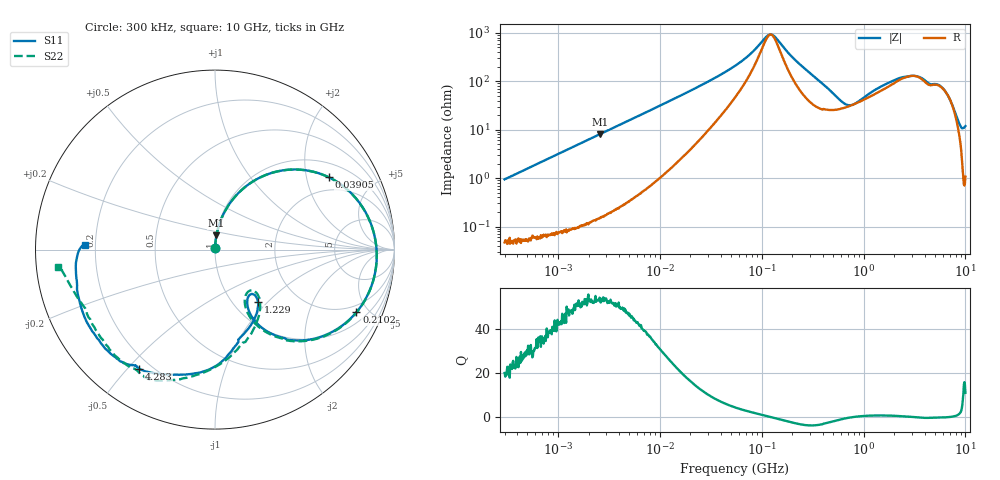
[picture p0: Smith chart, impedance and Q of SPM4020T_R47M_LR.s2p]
! S-Parameter Data Generated by TDK Corporation
! Copyright(C) 2019 TDK Corporation.
! All Rights Reserved.
! TDK P/N: SPM4020T-R47M-LR (Inductor)
! Property: L=470nH at 100kHz
! Size(LxWxT): 4.4x4.1x2mm
! Model Type: s2p (Touchstone File Format Version 1.0)
! Frequency: DC=Yes Start=0.3MHz Stop=10000MHz 802points Log-sweep
! Model Generated on Sep. 23, 2019
! Port Assignments:
!  1 ---@@@--- 2
! Applicable Conditions:
!  Temperature = 25 degC
!  DC Bias Current = 0 A
!  Small Signal Operation
! Terms and conditions regarding TDK Simulation Models
! (1)This simulation model is being provided solely for informational purposes. Please refer to the specifications of the products in terms of detailed characteristics of such products.
! (2)In no event shall TDK Corporation of any of its subsidiaries be liable for any loss or damage arising, directly or indirectly,
!  From any information contained in this simulation model, including, but not limited to loss or damages arising from any inaccuracies, omissions or errors in connection with such information.
! (3)Any and all copyrights on this simulation model are owned by TDK Corporation.
!  Duplication or redistribution of this simulation model without prior written permission from TDK Corporation is prohibited.
! (4)This simulation model is subject to any modification or change without any prior notice.
! (5)Neither TDK Corporation nor any of its subsidiaries shall make any warranty, express or implied,
!  Including but not limited to the correctness, implied warranties of merchantability and fitness for a particular purpose with respect to this simulation models.
! (6)The use of this simulation model shall be deemed to have consented to the terms and conditions hereof.
# Hz S MA R 50
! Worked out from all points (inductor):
!   801 points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, 300 kHz to 10 GHz, reference 50 ohm
!   read as one part in series: L = 498 nH near 318.3 kHz
!   highest Q = 53.8 at 2.599 MHz (marker M1), where L = 495 nH
!   self-resonance near 122.6 MHz
!   S11 on the Smith chart (normalised r, x): 300 kHz: 1.00, +0.02; 39.05 MHz: 1.47, +2.71; 210.2 MHz: 1.54, -4.19; 1.229 GHz: 1.29, -0.87; 4.283 GHz: 0.15, -0.54; 10 GHz: 0.16, +0.02
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300000  0.009137 86.2  0.9995 -0.6  0.9995 -0.5  0.009027 86.8
1713600  0.05275 85.8  0.9975 -3.1  0.9975 -3.1  0.05277 85.8
2598892  0.07965 84.2  0.9953 -4.7  0.9954 -4.7  0.07969 84.3
9671944  0.2837 71.4  0.9499 -16.8  0.95 -16.8  0.2836 71.4
2.252362e7  0.5639 50.9  0.787 -35.1  0.7871 -35.1  0.5639 50.9
3.904515e7  0.7508 32.5  0.564 -49.5  0.564 -49.5  0.7509 32.5
5.477226e7  0.8298 21.1  0.4024 -56.0  0.4024 -56.0  0.8298 21.0
1.210198e8  0.9025 -4.1  0.09762 -7.8  0.09765 -7.8  0.9025 -4.3
1.356511e8  0.9016 -7.8  0.1094 19.4  0.1095 19.4  0.9015 -8.1
2.102074e8  0.8619 -23.9  0.296 46.4  0.2961 46.4  0.8614 -24.4
3.126428e8  0.7506 -41.1  0.5083 35.0  0.5083 35.0  0.7489 -41.8
4.329008e8  0.5922 -54.4  0.6498 18.4  0.6499 18.4  0.5881 -55.3
6.242396e8  0.3991 -61.2  0.7282 -3.7  0.7283 -3.7  0.3878 -62.7
8.643532e8  0.3181 -52.9  0.7071 -23.9  0.7072 -23.9  0.299 -52.8
1.228555e9  0.3752 -50.6  0.6092 -45.6  0.6092 -45.6  0.3553 -46.9
1.767019e9  0.4839 -68.5  0.4438 -67.1  0.4438 -67.1  0.4872 -63.3
2.756092e9  0.6871 -96.4  0.2592 -80.0  0.2593 -80.0  0.6954 -96.6
3.472057e9  0.7512 -112.5  0.203 -76.1  0.2031 -76.1  0.7791 -110.5
4.282745e9  0.7868 -122.6  0.2089 -74.9  0.209 -75.0  0.8082 -120.4
6.41458e9  0.8235 -137.9  0.175 -96.0  0.175 -96.2  0.8019 -141.2
8.09931e9  0.8004 -163.8  0.1528 -114.9  0.1529 -115.0  0.8209 -163.6
1e10  0.7227 177.9  0.1167 -125.5  0.1167 -125.6  0.8788 -173.8
